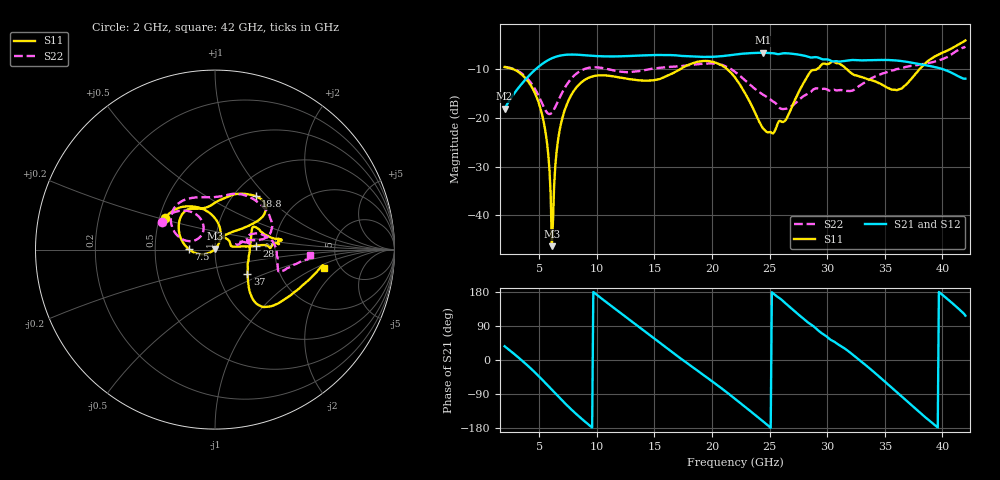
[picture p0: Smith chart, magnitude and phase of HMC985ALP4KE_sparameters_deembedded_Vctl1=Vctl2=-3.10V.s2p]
!s2p File: Measurements: S11, S21, S12, S22
# GHz S dB R 50.0
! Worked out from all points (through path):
!   401 points, 2 GHz to 42 GHz, reference 50 ohm
!   highest |S21| = -6.71 dB at 24.4 GHz (marker M1); lowest = -18.2 dB at 2 GHz (marker M2)
!   lowest |S11| = -46.3 dB at 6.1 GHz (marker M3), VSWR 1.01, Z = 50.1 + j0.476 ohm
!   |S11| at or under -10 dB: 2.657 GHz to 17.31 GHz (14.65 GHz wide, 147 % of centre); 21.29 GHz to 29.15 GHz (7.867 GHz wide, 31.2 % of centre); 31.67 GHz to 38.04 GHz (6.376 GHz wide, 18.3 % of centre)
!   |S22| runs from -19.3 to -5.5 dB; largest |S21 - S12| = 0.00049
!   S11 on the Smith chart (normalised r, x): 2 GHz: 0.54, +0.21; 7.5 GHz: 0.75, +0.00; 18.8 GHz: 1.25, +0.87; 28 GHz: 1.60, +0.07; 37 GHz: 1.38, -0.40; 42 GHz: 3.79, -1.24
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2  -9.63 147.2  -18.16 36.3  -18.16 36.2  -9.59 152.3
4.9  -16.53 83.6  -9.66 -40.8  -9.67 -40.8  -15.30 114.6
5.6  -23.73 62.8  -8.46 -62.5  -8.46 -62.5  -18.69 125.9
6.1  -46.31 79.3  -7.84 -78.5  -7.84 -78.5  -19.00 147.5
6.3  -33.82 -149.8  -7.65 -84.9  -7.65 -84.9  -18.27 154.6
6.7  -23.63 -157.3  -7.36 -97.6  -7.36 -97.6  -16.30 162.0
7.5  -16.72 179.1  -7.09 -122.1  -7.09 -122.1  -12.88 159.1
8.7  -12.70 150.6  -7.17 -155.5  -7.17 -155.5  -10.27 143.1
12.5  -11.97 115.4  -7.40 114.2  -7.40 114.1  -10.67 94.6
15.4  -12.13 95.0  -7.17 47.2  -7.18 47.1  -9.80 73.2
18.8  -8.53 52.8  -7.51 -29.6  -7.51 -29.6  -9.01 52.0
22  -11.77 34.3  -7.07 -102.4  -7.07 -102.4  -10.61 13.4
24.4  -22.08 64.2  -6.71 -161.1  -6.71 -161.1  -15.24 17.1
26.3  -20.71 12.5  -6.80 152.0  -6.80 152.0  -18.20 16.3
28  -12.71 5.5  -7.30 107.4  -7.30 107.3  -15.50 14.5
28.7  -10.27 1.7  -7.68 91.6  -7.68 91.6  -14.45 12.9
30.6  -8.59 7.6  -8.47 48.6  -8.48 48.5  -14.29 14.1
32.4  -11.30 22.5  -8.20 9.5  -8.20 9.5  -14.19 22.1
35.4  -14.03 8.2  -8.20 -67.7  -8.20 -67.7  -10.54 13.8
37  -12.88 -37.1  -8.59 -110.9  -8.60 -110.9  -9.53 4.3
39.5  -7.30 -47.5  -9.71 -175.5  -9.71 -175.6  -8.40 -18.6
42  -4.19 -9.4  -12.01 117.0  -12.02 117.0  -5.48 -3.1
